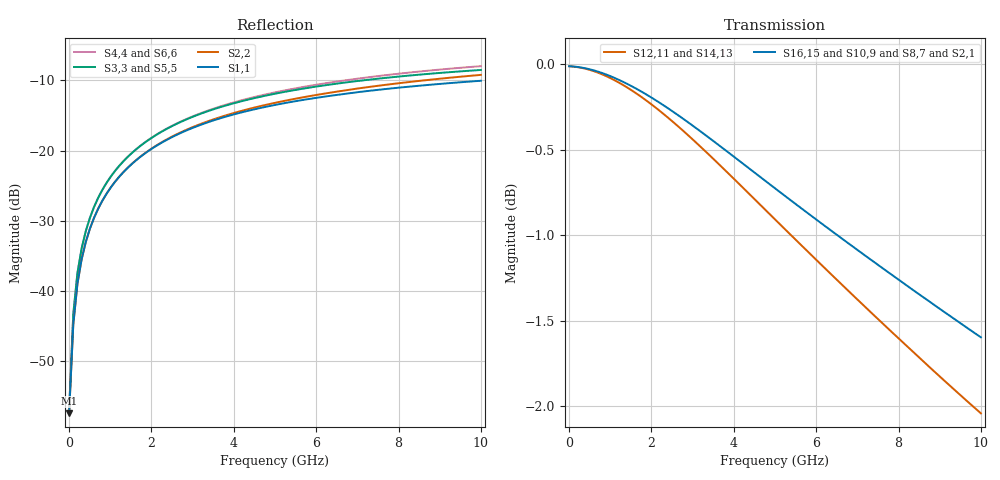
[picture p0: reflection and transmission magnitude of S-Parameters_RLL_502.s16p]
! Touchstone file written by nWave 4.6.3
! Mon Mar 11 14:47:17 2013
! Nimbic
! Project: SN65LVPE502A_RLL
! Simulation: APEX1
! User: a0220810
! Computer: dflcmp3924.dal.design.ti.com
! Single-ended  S-parameters
!NUMBER OF PORTS = 16
!  PORT#  PORT_NAME  NET_NAME
! PORT1:  10_BONDWIRE0.PIN050_GND 10
! PORT2:  10_Bot.PIN004_GND 10
! PORT3:  11_BONDWIRE0.PIN051_GND 11
! PORT4:  11_Bot.PIN003_GND 11
! PORT5:  19_BONDWIRE0.PIN039_GND 19
! PORT6:  19_Bot.PIN001_GND 19
! PORT7:  20_BONDWIRE0.PIN040_GND 20
! PORT8:  20_Bot.PIN002_GND 20
! PORT9:  22_BONDWIRE0.PIN042_GND 22
! PORT10:  22_Bot.PIN007_GND 22
! PORT11:  23_BONDWIRE0.PIN043_GND 23
! PORT12:  23_Bot.PIN008_GND 23
! PORT13:  7_BONDWIRE0.PIN047_GND 7
! PORT14:  7_Bot.PIN010_GND 7
! PORT15:  8_BONDWIRE0.PIN048_GND 8
! PORT16:  8_Bot.PIN009_GND 8
# HZ S RI R 50
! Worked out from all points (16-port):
!   100 points, 100 Hz to 10 GHz, reference 50 ohm
!   strongest paths, dB at 100 Hz, 2.525 GHz, 5.051 GHz, 7.576 GHz, 10 GHz:
!     S16,15: 0.0, -0.3, -0.7, -1.2, -1.6
!     S10,9: 0.0, -0.3, -0.7, -1.2, -1.6
!     S8,7: 0.0, -0.3, -0.8, -1.3, -1.7
!     S2,1: 0.0, -0.3, -0.8, -1.3, -1.8
!     S12,11: 0.0, -0.3, -0.9, -1.5, -2.0
!     S14,13: 0.0, -0.3, -0.9, -1.5, -2.1
!   lowest |S11| = -57.5 dB at 100 Hz (marker M1), VSWR 1.00, Z = 50.1 - j1.56e-06 ohm
!   |S11| at or under -10 dB: start of sweep to end of sweep
